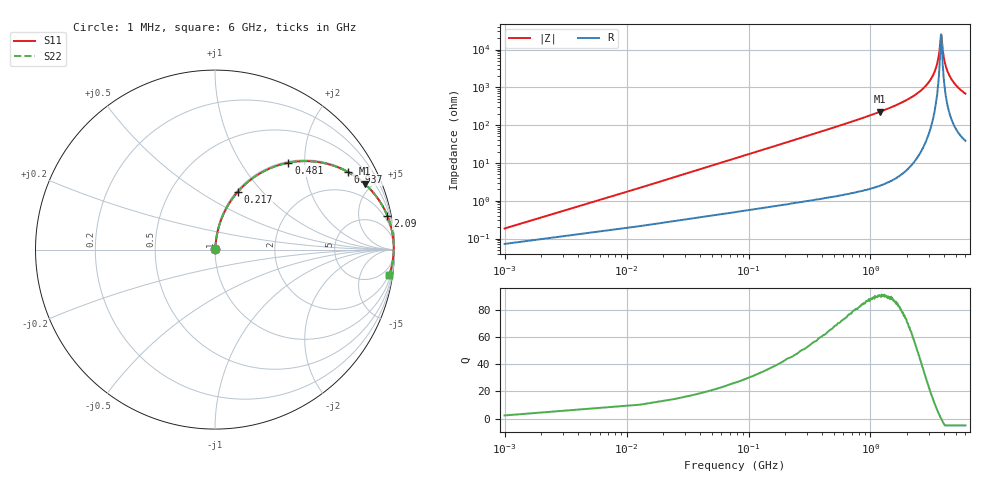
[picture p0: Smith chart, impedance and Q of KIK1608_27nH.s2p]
!version-2
!date-01.2022
!Series
# MHz S RI R 50
!Freq ReS11 ImS11 ReS21 ImS21 ReS12 ImS12 ReS22 ImS22
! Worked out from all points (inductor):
!   501 points, 1 MHz to 6 GHz, reference 50 ohm
!   read as one part in series: L = 27 nH near 25 MHz
!   highest Q = 90.5 at 1.2 GHz (marker M1), where L = 30 nH
!   self-resonance near 3.79 GHz
!   S11 on the Smith chart (normalised r, x): 1 MHz: 1.00, +0.00; 217 MHz: 1.02, +0.74; 481 MHz: 1.03, +1.66; 937 MHz: 1.04, +3.39; 2.09 GHz: 1, +10; 6 GHz: 2, -14
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1  0.000743 0.00169  0.9993 -0.00169  0.9993 -0.00169  0.000743 0.00169
37  0.00737 0.0621  0.9926 -0.0621  0.9926 -0.0621  0.00737 0.0621
61  0.0149 0.1015  0.9851 -0.1015  0.9851 -0.1015  0.0149 0.1015
121  0.0459 0.1948  0.9541 -0.1948  0.9541 -0.1948  0.0459 0.1948
217  0.1255 0.3203  0.8745 -0.3203  0.8745 -0.3203  0.1255 0.3203
481  0.4089 0.4841  0.5911 -0.4841  0.5911 -0.4841  0.4089 0.4841
937  0.7389 0.4335  0.2611 -0.4335  0.2611 -0.4335  0.7389 0.4335
1010  0.7698 0.4153  0.2302 -0.4153  0.2302 -0.4153  0.7698 0.4153
1200  0.834 0.3666  0.166 -0.3666  0.166 -0.3666  0.834 0.3666
2020  0.9552 0.1998  0.0448 -0.1998  0.0448 -0.1998  0.9552 0.1998
2090  0.9601 0.1884  0.0399 -0.1884  0.0399 -0.1884  0.9601 0.1884
3010  0.9917 0.0717  0.00831 -0.0717  0.00831 -0.0717  0.9917 0.0717
3520  0.9958 0.0237  0.00419 -0.0237  0.00419 -0.0237  0.9958 0.0237
3640  0.9961 0.0133  0.00394 -0.0133  0.00394 -0.0133  0.9961 0.0133
3790  0.996 0.000396  0.00397 -0.000396  0.00397 -0.000396  0.996 0.000396
3820  0.996 -0.00154  0.004 0.00154  0.004 0.00154  0.996 -0.00154
3920  0.9957 -0.0101  0.00425 0.0101  0.00425 0.0101  0.9957 -0.0101
4010  0.9954 -0.0166  0.00455 0.0166  0.00455 0.0166  0.9954 -0.0166
4160  0.9947 -0.0284  0.00532 0.0284  0.00532 0.0284  0.9947 -0.0284
4400  0.993 -0.0456  0.007 0.0456  0.007 0.0456  0.993 -0.0456
5010  0.9866 -0.085  0.0134 0.085  0.0134 0.085  0.9866 -0.085
6000  0.9711 -0.1414  0.0289 0.1414  0.0289 0.1414  0.9711 -0.1414
